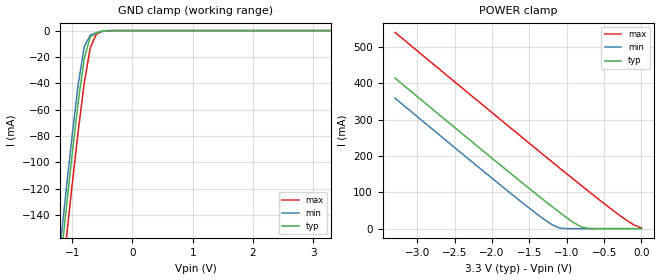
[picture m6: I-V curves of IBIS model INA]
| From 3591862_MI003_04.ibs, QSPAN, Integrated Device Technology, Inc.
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|   Model INA
[Model]   INA
Model_type   Input
Polarity   Non-Inverting
Vinl =   0.8000V
Vinh =   2.0000V
C_comp   5.00pF   5.00pF   5.00pF
[Voltage Range]   3.3000V   3.0000V   4.0000V
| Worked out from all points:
|   GND clamp passes 1 mA (typ) near -0.54 V on its own axis
|   POWER clamp passes 1 mA (typ) near -0.72 V on its own axis
[GND_clamp]
| voltage   I(typ)   I(min)   I(max)
-3.3V     -1.142A    -1.129A    -1.164A
-1.2V     -178.9mA   -164.2mA   -202.5mA
-1.1V     -135.5mA   -120.9mA   -159.1mA
-1V       -93.44mA   -79.05mA   -116.7mA
-900mV    -53.99mA   -40.63mA   -76.27mA
-800mV    -21.15mA   -12.18mA   -39.75mA
-700mV    -4.899mA   -3.529mA   -12.96mA
-600mV    -1.729mA   -1.656mA   -2.71mA
-500mV    -436.8uA   -367.2uA   -593.5uA
-400mV    -40.4uA    -22.34uA   -82.77uA
3.3V      128.4pA    114.1pA    315.7pA
[POWER_clamp]
| voltage   I(typ)   I(min)   I(max)
-3.3V     414.6mA    359.3mA    540.4mA
-1.8V     160.3mA    105.4mA    285.5mA
-1.4V     93.75mA    40.4mA     218.1mA
-1.2V     61.21mA    11.22mA    184.5mA
-1.1V     45.35mA    1.83mA     167.8mA
-900mV    15.71mA    7.867uA    134.5mA
-800mV    4.379mA    260.1nA    118mA
-700mV    364.3uA    7.423nA    101.6mA
-200mV    236pA      111.7pA    23.19mA
-100mV    134.6pA    109.2pA    10.25mA
0V        128.4pA    106.8pA    1.957mA
